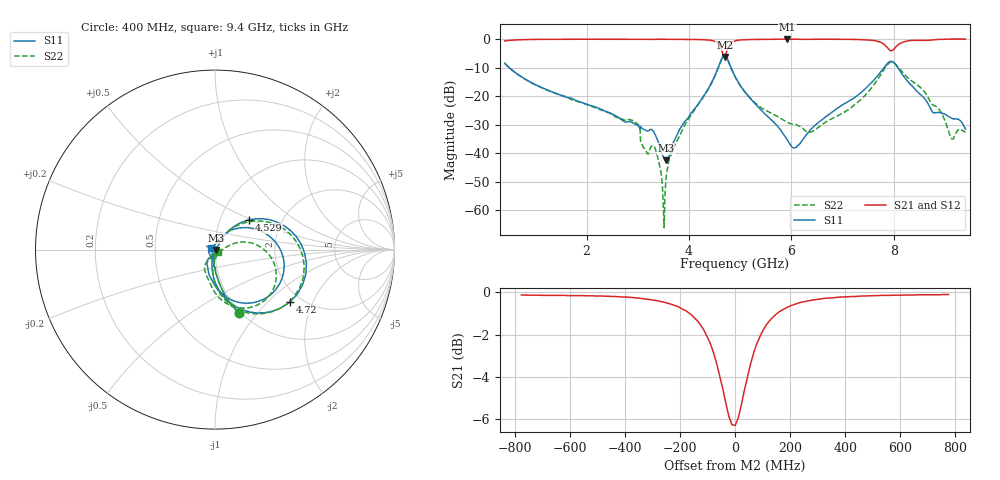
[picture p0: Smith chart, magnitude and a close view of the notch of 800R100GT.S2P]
!  American Technical Ceramics  Date:  6/19/09
!  One Norden Lane
!  Huntington Station,  NY.  11746-2102
!  Tel:  (631) 622-4700  Fax:  (631) 622-4748
!  Part Number  800R100GT
!  Description: Ultra-low ESR, NPO  Mounting Orientation: Horizontal
!  Application: High RF power Filters, Combiners, Matching networks,
!  Antenna, DC block, Bypass and Couplers
# GHZ S DB R 50
! Freq  |S11|  S11 Ph  |S21|  S21 Ph  |S12|  S12 Ph  |S22|  S22 Ph
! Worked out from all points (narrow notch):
!   801 points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, 400 MHz to 9.4 GHz, reference 50 ohm
!   highest |S21| = -0.01 dB at 5.924 GHz (marker M1); lowest = -6.3 dB at 4.698 GHz (marker M2)
!   notch at M2: 6.2 dB deep, 131 MHz wide at half that depth
!   lowest |S11| = -42.5 dB at 3.55 GHz (marker M3), VSWR 1.02, Z = 50.7 - j0.19 ohm
!   |S11| at or under -10 dB: 488.8 MHz to 4.571 GHz (4.083 GHz wide, 161 % of centre); 4.821 GHz to 7.812 GHz (2.99 GHz wide, 47.3 % of centre); 8.08 GHz to end of sweep
!   |S22| runs from -66.1 to -5.7 dB; largest |S21 - S12| = 0.0036
!   S11 on the Smith chart (normalised r, x): 400 MHz: 0.98, -0.81; 4.529 GHz: 1.37, +0.49; 4.72 GHz: 1.74, -1.37; 9.4 GHz: 0.95, +0.02
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0.4  -8.46 -69.6  -0.68 20.2  -0.69 20.3  -8.48 -69.5
1.908  -22.23 -93.7  -0.06 -4.4  -0.07 -4.3  -22.34 -92.9
2.954  -29.88 -101.6  -0.07 -11.4  -0.07 -11.3  -29.16 -92.2
3.145  -31.94 -70.2  -0.08 -12.8  -0.09 -12.7  -38.85 -91.4
3.404  -36.21 -71.9  -0.06 -14.2  -0.07 -14.1  -42.40 -86.6
3.494  -41.14 -44.6  -0.06 -15.0  -0.07 -14.9  -56.04 -81.0
3.55  -42.46 -14.4  -0.06 -15.5  -0.07 -15.3  -49.44 59.1
3.606  -41.12 15.1  -0.08 -15.9  -0.08 -15.8  -42.74 58.1
3.73  -34.92 43.9  -0.09 -16.9  -0.09 -16.8  -36.99 61.7
4.529  -11.92 40.9  -0.97 -32.3  -0.97 -32.2  -12.13 38.9
4.698  -5.58 -21.9  -6.30 -15.8  -6.30 -15.7  -5.72 -24.3
4.72  -5.87 -35.1  -5.37 -4.2  -5.37 -4.0  -6.01 -37.6
4.9  -13.07 -84.9  -0.64 -7.9  -0.64 -7.8  -13.23 -86.8
5.924  -35.40 -151.5  -0.01 -23.0  -0.01 -22.9  -29.17 -74.3
6.093  -37.97 152.3  -0.06 -24.6  -0.06 -24.4  -30.05 -64.1
6.408  -31.23 90.7  -0.09 -26.2  -0.08 -26.0  -32.45 -30.4
7.353  -18.91 55.3  -0.19 -34.7  -0.18 -34.5  -21.30 16.5
7.904  -8.11 -11.5  -3.58 -41.1  -3.57 -41.0  -8.50 -24.9
8.241  -14.17 -90.9  -0.77 -23.7  -0.76 -23.5  -13.00 -92.6
8.883  -25.72 -113.8  -0.12 -31.2  -0.11 -31.0  -24.58 -118.9
9.13  -27.71 -127.9  -0.01 -32.8  -0.01 -32.7  -34.84 -88.2
9.4  -31.61 158.7  -0.01 -35.4  -0.01 -35.2  -32.58 -34.8
